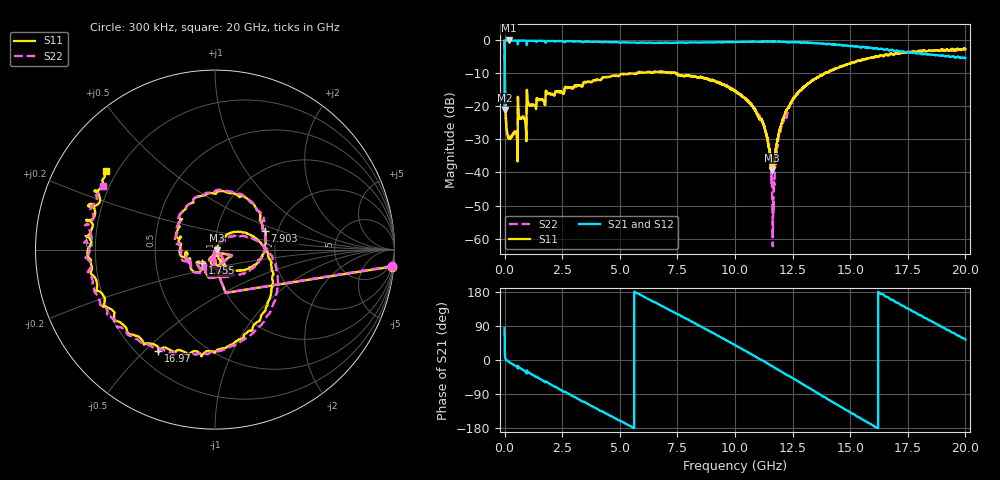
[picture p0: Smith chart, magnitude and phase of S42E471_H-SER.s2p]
!{S42E471}
!Johanson Technology Inc.
!www.johansontechnology.com
!Test Board Conditions:
!Substrate Type  RO4350B
!Substrate Thickness  50 mil
!Substrate Dk  3.66
!TL Type: GCPW
!TL Trace Width  60 mil
!TL Gap  10 mil
!Electrode orientation  Horizontal
!DUT TOPOLOGY	SERIES
!Mounting Pad LxW  14x55 mil
! Created Wed Nov 25 22:18:24 2020
# khz S ma R 50
! 2 Port Network Data from SP1.SP block
! freq  magS11  angS11  magS21  angS21  magS12  angS12  magS22  angS22
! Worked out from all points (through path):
!   20001 points, 300 kHz to 20 GHz, reference 50 ohm
!   highest |S21| = -0.01 dB at 192.3 MHz (marker M1); lowest = -21.1 dB at 300 kHz (marker M2)
!   group delay of S21, straight-line fit = 93.2 ps
!   lowest |S11| = -39.2 dB at 11.62 GHz (marker M3), VSWR 1.02, Z = 51 - j0.38 ohm
!   |S11| at or under -10 dB: 10.21 MHz to 5.458 GHz (5.448 GHz wide, 199 % of centre); 5.517 GHz to 5.75 GHz (232.6 MHz wide, 4.13 % of centre); 7.499 GHz to 13.89 GHz (6.394 GHz wide, 59.8 % of centre)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
!   |S22| runs from -62.3 to -0.1 dB; largest |S21 - S12| = 0.015
!   S11 on the Smith chart (normalised r, x): 300 kHz: 2, -21; 1.755 GHz: 0.85, -0.13; 7.903 GHz: 1.72, +0.39; 16.97 GHz: 0.29, -0.55; 20 GHz: 0.16, +0.31
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300  0.9904 -5.5  0.08822 84.3  0.08777 84.1  0.9913 -5.3
101300  0.04142 -91.1  0.9978 -1.4  0.999 -1.5  0.04208 -91.3
192300  0.033 -96.1  0.9993 -5.4  0.9971 -5.3  0.03379 -96.3
854300  0.06612 -120.2  0.9951 -28.3  0.995 -28.3  0.06878 -116.3
1055300  0.1057 -125.2  0.9909 -33.4  0.9914 -33.4  0.1082 -121.2
1755300  0.1047 -134.2  0.9601 -59.0  0.9603 -59.0  0.105 -132.3
3334300  0.2035 159.1  0.9613 -108.0  0.9616 -108.0  0.1991 168.7
4865300  0.29 115.3  0.9425 -156.1  0.9428 -156.1  0.291 115.3
6667300  0.3348 56.8  0.923 147.8  0.9225 147.7  0.3383 60.3
7903300  0.2977 20.5  0.9244 108.5  0.9239 108.7  0.2965 20.0
8859300  0.2565 -11.8  0.9344 77.2  0.9354 77.1  0.2591 -13.3
1.00003e7  0.1723 -43.5  0.9475 39.4  0.947 39.4  0.1757 -55.5
1.11943e7  0.05882 -65.6  0.9556 -1.2  0.954 -1.2  0.05788 -101.8
1.14303e7  0.02919 -63.4  0.961 -9.7  0.9608 -9.7  0.02794 -113.4
1.16153e7  0.01094 -19.9  0.9605 -16.3  0.9606 -16.3  0.004196 -110.7
1.20803e7  0.06386 58.5  0.9554 -33.2  0.955 -33.2  0.05823 45.4
1.33343e7  0.2426 12.6  0.917 -78.3  0.9181 -78.3  0.2438 10.7
1.50373e7  0.4529 -55.7  0.8217 -140.0  0.8243 -139.8  0.4545 -46.6
1.66673e7  0.5936 -107.9  0.7105 164.6  0.7139 163.8  0.6073 -105.8
1.69723e7  0.6454 -119.2  0.6952 152.3  0.7027 153.0  0.6282 -115.4
1.84463e7  0.7053 -169.2  0.6145 104.5  0.6161 104.9  0.7042 -159.1
2e7  0.7475 144.3  0.5418 54.0  0.5424 54.4  0.724 150.3
